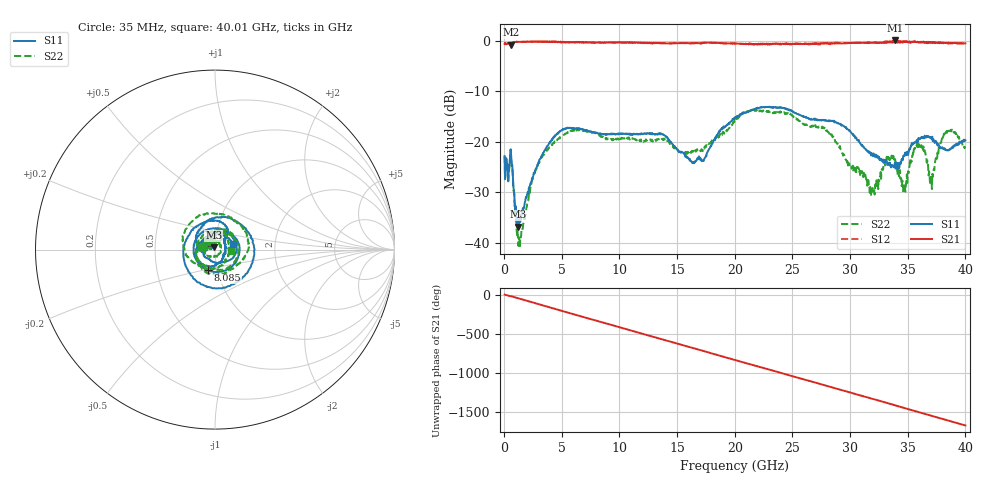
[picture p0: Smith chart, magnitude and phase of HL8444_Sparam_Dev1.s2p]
! 1/27/2023 9:40:07 AM
! D:\SMA SENSE\127\FIN\SN1.S2P
! CHANNEL.1
! TR.MEASUREMENT
! CORRECTED.DATA
# GHZ S RI R 50.0
! FREQ.GHZ  S11RE  S11IM  S21RE  S21IM  S12RE  S12IM  S22RE  S22IM
!; PortSelection: Port_12
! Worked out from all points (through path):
!   1143 points, 35 MHz to 40.01 GHz, reference 50 ohm
!   highest |S21| = 0.01 dB at 33.91 GHz (marker M1); lowest = -0.8 dB at 560 MHz (marker M2)
!   group delay of S21, straight-line fit = 116 ps
!   lowest |S11| = -36.8 dB at 1.225 GHz (marker M3), VSWR 1.03, Z = 49.3 + j1.27 ohm
!   |S11| at or under -10 dB: start of sweep to end of sweep
!   |S22| runs from -40.6 to -13.5 dB; largest |S21 - S12| = 0.049
!   S11 on the Smith chart (normalised r, x): 35 MHz: 0.87, +0.03; 8.085 GHz: 0.90, -0.21; 40.01 GHz: 1.22, +0.07
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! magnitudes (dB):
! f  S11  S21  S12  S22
! 35 MHz  -22.9  -0.7  -0.7  -22.8
! 560 MHz  -21.5  -0.8  -0.9  -21.7
! 1.225 GHz  -36.8  -0.3  -0.2  -40.6
! 3.255 GHz  -22.7  -0.3  -0.3  -23.0
! 4.935 GHz  -17.8  -0.4  -0.3  -18.9
! 6.72 GHz  -17.5  -0.4  -0.3  -17.8
! 8.085 GHz  -18.3  -0.4  -0.4  -18.5
! 13.37 GHz  -18.4  -0.5  -0.5  -19.4
! 16.48 GHz  -24.2  -0.5  -0.5  -21.9
! 20.02 GHz  -15.2  -0.6  -0.6  -15.6
! 21.8 GHz  -13.6  -0.7  -0.8  -13.7
! 26.7 GHz  -15.6  -0.6  -0.6  -16.8
! 28.39 GHz  -15.9  -0.5  -0.7  -18.7
! 31.95 GHz  -22.8  -0.4  -0.3  -29.4
! 33.35 GHz  -24.3  -0.4  -0.3  -23.1
! 33.91 GHz  -24.1  0.0  -0.1  -23.5
! 34.65 GHz  -22.8  -0.3  -0.2  -29.9
! 35.88 GHz  -20.0  -0.2  -0.3  -21.0
! 36.44 GHz  -19.0  -0.5  -0.2  -21.6
! 36.99 GHz  -19.0  -0.3  -0.3  -27.0
! 38.29 GHz  -21.5  -0.5  -0.5  -18.6
! 40.01 GHz  -19.7  -0.6  -0.6  -21.0
